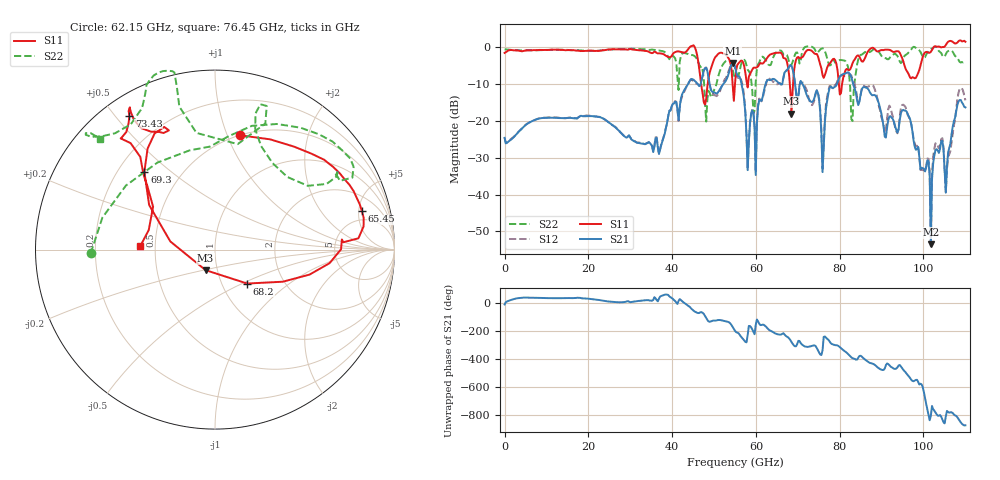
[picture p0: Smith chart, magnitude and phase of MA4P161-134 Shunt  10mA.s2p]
!Keysight Technologies,N5247B,US61255204,A.15.70.20
!Date: Friday, October 21, 2022 14:13:56
!Correction: S11(C  4-Port  )
!S31(C  4-Port  )
!S13(C  4-Port  )
!S33(C  4-Port  )
!S2P File: Measurements: S11, S31, S13, S33:
# Hz S  dB  R 50
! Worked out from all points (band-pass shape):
!   401 points, 10 MHz to 110 GHz, reference 50 ohm
!   highest |S21| = -4.28 dB at 54.46 GHz (marker M1); lowest = -53.6 dB at 101.8 GHz (marker M2)
!   |S21| within 3 dB of the highest: 53.46 GHz to 55.44 GHz (1.986 GHz wide, 3.65 % of centre); 66.75 GHz to 69.02 GHz (2.275 GHz wide, 3.35 % of centre)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
!   lowest |S11| = -18.0 dB at 68.48 GHz (marker M3), VSWR 1.29, Z = 43.9 - j10.2 ohm
!   |S11| at or under -10 dB: 46.93 GHz to 48.49 GHz (1.556 GHz wide, 3.26 % of centre); 54.45 GHz to 55 GHz (556.7 MHz wide, 1.02 % of centre); 68.09 GHz to 68.86 GHz (771.7 MHz wide, 1.13 % of centre)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
!   |S22| runs from -20.2 to 0.3 dB; largest |S21 - S12| = 0.16
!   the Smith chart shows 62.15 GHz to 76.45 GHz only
!   S11 on the Smith chart (normalised r, x): 62.15 GHz: 0.50, +1.11; 65.45 GHz: 3.61, +5.43; 68.2 GHz: 1.31, -0.53; 69.3 GHz: 0.31, +0.41; 73.43 GHz: 0.08, +0.54; 76.45 GHz: 0.41, +0.02
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1e7  -1.52 -179.2  -24.59 -13.0  -24.57 -12.5  -0.64 -179.3
1.843332e10  -0.99 130.6  -18.64 30.9  -18.65 30.7  -0.84 140.4
3.685665e10  -1.63 126.2  -28.99 29.0  -28.86 29.0  -0.88 133.7
4.565585e10  -0.72 52.1  -9.40 -68.1  -9.77 -66.6  -2.73 27.0
5.445505e10  -10.13 98.2  -4.28 -174.2  -4.34 -174.1  -5.96 127.6
5.5005e10  -9.97 -177.2  -5.32 158.6  -5.53 158.1  -8.28 148.1
5.802972e10  -10.91 159.6  -33.37 128.5  -33.16 127.2  -6.12 167.4
6.077948e10  -4.68 149.3  -14.31 -149.7  -13.95 -150.8  -4.16 -121.8
6.215435e10  -3.72 77.8  -10.53 -165.0  -11.24 -159.6  -3.19 -178.3
6.545405e10  -1.46 14.7  -9.68 132.1  -9.69 153.8  -0.92 37.9
6.82038e10  -11.68 -46.5  -4.79 93.1  -4.95 90.0  -4.87 45.1
6.847878e10  -18.00 -114.5  -4.98 79.7  -5.17 77.3  -4.75 56.5
6.93037e10  -4.65 132.3  -9.57 48.1  -9.30 47.3  -2.03 73.4
7.342832e10  -1.05 122.6  -14.87 51.7  -15.71 49.7  0.11 111.0
7.645305e10  -7.58 177.6  -20.45 118.2  -19.43 130.1  -1.02 136.0
8.085265e10  -8.20 -75.6  -7.23 20.8  -7.65 21.1  -3.50 -144.2
8.305245e10  -4.36 -45.6  -9.32 -36.7  -8.78 -20.7  -20.04 12.6
8.607718e10  -2.79 6.4  -10.87 -47.2  -10.72 -46.2  -1.28 -14.8
9.185165e10  -0.68 71.5  -18.78 -86.1  -15.84 -83.3  -3.00 67.2
9.762612e10  -8.23 177.9  -25.25 158.6  -24.77 156.7  0.15 165.9
1.017508e11  -1.22 -88.0  -53.58 -87.9  -54.04 -80.1  -0.51 -124.6
1.1e11  1.51 8.0  -16.33 -156.1  -14.40 -161.6  -4.06 16.5
